| / 7\'7
| \ \   Xilinx Inc.
| / /
| \_\/.\   IBIS Models for Virtex-II
[IBIS ver]   2.1
[File name]   virtex2.ibs
[File Rev]   3.1
[Date]   6/8/04
[Source]   HSPICE simulations
[Notes]   Xilinx IBIS models for Virtex-II I/Os
These models have been verified to be an accurate representation of the
FAST/STRONG, SLOW/WEAK and TYPICAL performance corners by sample testing
of actual devices.  Actual measurements may vary, but will be well within
the performance corners if the simulation includes all other elements
that are on the printed circuit board.  These include but are not limited
to: driver, receiver(s), transmission line(s), connectors, impedance
discontinuities, and package parasitics.  Contact your Xilinx FAE or the
Xilinx Hotline for assistance.
For more information about using these IBIS models, please see
the readme file that came with this model file.
[Copyright]   Copyright 2003, Xilinx Inc., All rights reserved
|   Component Virtex-II
[Component]   Virtex-II
[Manufacturer]   Xilinx Inc.
[Package]
| variable   typ   min   max
R_pkg   0.1   NA   NA
L_pkg   0.8nH   NA   NA
C_pkg   0.5pF   NA   NA
[Pin]  signal_name   model_name   R_pin   L_pin   C_pin
|   LVTTL, fast slew rate
1   LVTTL2F   LVTTL2F
2   LVTTL4F   LVTTL4F
3   LVTTL6F   LVTTL6F
4   LVTTL8F   LVTTL8F
5   LVTTL12F   LVTTL12F
6   LVTTL16F   LVTTL16F
7   LVTTL24F   LVTTL24F
|   LVTTL, slow slew rate
8   LVTTL2S   LVTTL2S
9   LVTTL4S   LVTTL4S
10   LVTTL6S   LVTTL6S
11   LVTTL8S   LVTTL8S
12   LVTTL12S   LVTTL12S
13   LVTTL16S   LVTTL16S
14   LVTTL24S   LVTTL24S
|   LVCMOS 3.3V, fast slew rate
15   LVCM32F   LVCM32F
16   LVCM34F   LVCM34F
17   LVCM36F   LVCM36F
18   LVCM38F   LVCM38F
19   LVCM312F   LVCM312F
20   LVCM316F   LVCM316F
21   LVCM324F   LVCM324F
|   LVCMOS 3.3V, slow slew rate
22   LVCM32S   LVCM32S
23   LVCM34S   LVCM34S
24   LVCM36S   LVCM36S
25   LVCM38S   LVCM38S
26   LVCM312S   LVCM312S
27   LVCM316S   LVCM316S
28   LVCM324S   LVCM324S
|   LVCMOS 2.5V, fast slew rate
29   LVCM22F   LVCM22F
30   LVCM24F   LVCM24F
31   LVCM26F   LVCM26F
32   LVCM28F   LVCM28F
33   LVCM212F   LVCM212F
34   LVCM216F   LVCM216F
35   LVCM224F   LVCM224F
|   LVCMOS 2.5V, slow slew rate
36   LVCM22S   LVCM22S
37   LVCM24S   LVCM24S
38   LVCM26S   LVCM26S
39   LVCM28S   LVCM28S
40   LVCM212S   LVCM212S
41   LVCM216S   LVCM216S
42   LVCM224S   LVCM224S
|   LVCMOS 1.8V, fast slew rate
43   LVCM82F   LVCM82F
44   LVCM84F   LVCM84F
45   LVCM86F   LVCM86F
46   LVCM88F   LVCM88F
47   LVCM812F   LVCM812F
48   LVCM816F   LVCM816F
|   LVCMOS 1.8V, slow slew rate
49   LVCM82S   LVCM82S
50   LVCM84S   LVCM84S
51   LVCM86S   LVCM86S
52   LVCM88S   LVCM88S
53   LVCM812S   LVCM812S
54   LVCM816S   LVCM816S
|   LVCMOS 1.5V, fast slew rate
55   LVCM52F   LVCM52F
56   LVCM54F   LVCM54F
57   LVCM56F   LVCM56F
58   LVCM58F   LVCM58F
59   LVCM512F   LVCM512F
60   LVCM516F   LVCM516F
|   LVCMOS 1.5V, slow slew rate
61   LVCM52S   LVCM52S
62   LVCM54S   LVCM54S
63   LVCM56S   LVCM56S
64   LVCM58S   LVCM58S
65   LVCM512S   LVCM512S
66   LVCM516S   LVCM516S
|   HSTL 1.5V, class I-IV
67   HSTL1_15   HSTL1_15
68   HSTL2_15   HSTL2_15
69   HSTL3_15   HSTL3_15
70   HSTL4_15   HSTL4_15
|   GTL, GTLP
71   GTL   GTL
72   GTLP   GTLP
|   SSTL 1.8V, class I and II
73   SSTL18C1   SSTL18C1
74   SSTL18C2   SSTL18C2
|   SSTL2, class I and II
75   SSTL2C1   SSTL2C1
76   SSTL2C2   SSTL2C2
|   SSTL3, class I and II
77   SSTL3C1   SSTL3C1
78   SSTL3C2   SSTL3C2
|   PCI
79   PCI33   PCI33
80   PCI66   PCI66
81   PCIX   PCIX
|   AGP
82   AGP2X   AGP2X
|   LVPECL
83P   LVPECLP   LVPECL
83N   LVPECLN   LVPECL
|   LVDS 2.5V
84P   LVDS25P   LVDS25
84N   LVDS25N   LVDS25
|   LVDS 2.5V Extended
85P   LVDS25EP   LVDS25E
85N   LVDS25EN   LVDS25E
|   LVDS 3.3V
86P   LVDS33P   LVDS33
86N   LVDS33N   LVDS33
|   LVDS 3.3V Extended
87P   LVDS33EP   LVDS33E
87N   LVDS33EN   LVDS33E
|   LDT 2.5V
88P   LDT25P   LDT25
88N   LDT25N   LDT25
|   BusLVDS
89P   BUSSLVDSP   BUSSLVDS
89N   BUSSLVDSN   BUSSLVDS
|   DCI HSTL 1.5V, class I-IV, inputs
90   DCIHSTL15_I   DCIHSTL15_I
91   DCIHSTL25_I   DCIHSTL25_I
92   DCIHSTL35_I   DCIHSTL35_I
93   DCIHSTL45_I   DCIHSTL45_I
|   DCI HSTL 1.5V, class I-IV, outputs
94   DCIHSTL15_O   DCIHSTL15_O
95   DCIHSTL25_O   DCIHSTL25_O
96   DCIHSTL35_O   DCIHSTL35_O
97   DCIHSTL45_O   DCIHSTL45_O
|   DCI GTL and GTLP, inputs
98   DCIGTL_I   DCIGTL_I
99   DCIGTLP_I   DCIGTLP_I
|   DCI GTL and GTLP, outputs
100   DCIGTL_O   DCIGTL_O
101   DCIGTLP_O   DCIGTLP_O
|   DCI SSTL 1.8V, class I and II, inputs
102   DCISSTL18C1_I   DCISSTL18C1_I
103   DCISSTL18C2_I   DCISSTL18C2_I
|   DCI SSTL2, class I and II, inputs
104   DCISSTL2C1_I   DCISSTL2C1_I
105   DCISSTL2C2_I   DCISSTL2C2_I
|   DCI SSTL3, class I and II, inputs
106   DCISSTL3C1_I   DCISSTL3C1_I
107   DCISSTL3C2_I   DCISSTL3C2_I
|   DCI SSTL 1.8V, class I and II, outputs
108   DCISSTL18C1_O   DCISSTL18C1_O
109   DCISSTL18C2_O   DCISSTL18C2_O
|   DCI SSTL2, class I and II, outputs
110   DCISSTL2C1_O   DCISSTL2C1_O
111   DCISSTL2C2_O   DCISSTL2C2_O
|   DCI SSTL3, class I and II, outputs
112   DCISSTL3C1_O   DCISSTL3C1_O
113   DCISSTL3C2_O   DCISSTL3C2_O
|   DCI LVCMOS 1.5V (40, 50, 65 ohms)
114   DCILVCMOS15_40   DCILVCMOS15_40
115   DCILVCMOS15_50   DCILVCMOS15_50
116   DCILVCMOS15_65   DCILVCMOS15_65
|   DCI LVCMOS 1.8V (40, 50, 65 ohms)
117   DCILVCMOS18_40   DCILVCMOS18_40
118   DCILVCMOS18_50   DCILVCMOS18_50
119   DCILVCMOS18_65   DCILVCMOS18_65
|   DCI LVCMOS 2.5V (40, 50, 65 ohms)
120   DCILVCMOS25_40   DCILVCMOS25_40
121   DCILVCMOS25_50   DCILVCMOS25_50
122   DCILVCMOS25_65   DCILVCMOS25_65
|   DCI LVCMOS 3.3V (40, 50, 65 ohms)
123   DCILVCMOS33_40   DCILVCMOS33_40
124   DCILVCMOS33_50   DCILVCMOS33_50
125   DCILVCMOS33_65   DCILVCMOS33_65
|   DCI LVCMOS 1.5V - 3.3V, DV2 drivers
|   (*DV2_50 = 25 ohms, *DV2_65 = 32.5 ohms)
126   DCILVCMOS15DV2_50   DCILVCMOS15DV2_50
127   DCILVCMOS15DV2_65   DCILVCMOS15DV2_65
128   DCILVCMOS18DV2_50   DCILVCMOS18DV2_50
129   DCILVCMOS18DV2_65   DCILVCMOS18DV2_65
130   DCILVCMOS25DV2_50   DCILVCMOS25DV2_50
131   DCILVCMOS25DV2_65   DCILVCMOS25DV2_65
132   DCILVCMOS33DV2_50   DCILVCMOS33DV2_50
133   DCILVCMOS33DV2_65   DCILVCMOS33DV2_65
|   HSTL 1.8V, class I-IV
134   HSTL1_18   HSTL1_18
135   HSTL2_18   HSTL2_18
136   HSTL3_18   HSTL3_18
137   HSTL4_18   HSTL4_18
|   DCI HSTL 1.8V, class I-IV, inputs
138   DCIHSTL18_I   DCIHSTL18_I
139   DCIHSTL28_I   DCIHSTL28_I
140   DCIHSTL38_I   DCIHSTL38_I
141   DCIHSTL48_I   DCIHSTL48_I
|   DCI HSTL 1.8V, class I-IV, outputs
142   DCIHSTL18_O   DCIHSTL18_O
143   DCIHSTL28_O   DCIHSTL28_O
144   DCIHSTL38_O   DCIHSTL38_O
145   DCIHSTL48_O   DCIHSTL48_O
|   LVDS 2.5V input, DCI-controlled termination
146   DCILVDS25   DCILVDS25
|   High-Speed LVDCI (1.8V DCI LVCMOS driver, HSTL1 receiver)
|   40, 50, 65 ohms
|   *DV2_50 = 25 ohms, *DV2_65 = 32.5 ohms
147   HSLVDCI_18_40   HSLVDCI_18_40
148   HSLVDCI_18_50   HSLVDCI_18_50
149   HSLVDCI_18_65   HSLVDCI_18_65
150   HSLVDCI_18_DV2_50   HSLVDCI_18_DV2_50
151   HSLVDCI_18_DV2_65   HSLVDCI_18_DV2_65
PGND   GND   GND
VCCO   VCCO   POWER
[Diff Pin]   inv_pin   vdiff   tdelay_typ   tdelay_min   tdelay_max
| Here is just a sample format for differential pin pairs.
| Edit the list based on your applications.
83P   83N   850mV   0   0   0
84P   84N   350mV   0   0   0
85P   85N   630mV   0   0   0
86P   86N   350mV   0   0   0
87P   87N   630mV   0   0   0
88P   88N   600mV   0   0   0
89P   89N   350mV   0   0   0
| Models and submodels in the file (151): LVTTL2F (I/O), LVTTL4F (I/O), LVTTL6F (I/O), LVTTL8F (I/O), LVTTL12F (I/O), LVTTL16F (I/O), LVTTL24F (I/O), LVTTL2S (I/O), LVTTL4S (I/O), LVTTL6S (I/O), LVTTL8S (I/O), LVTTL12S (I/O), LVTTL16S (I/O), LVTTL24S (I/O), LVCM32F (I/O), LVCM34F (I/O), LVCM36F (I/O), LVCM38F (I/O), LVCM312F (I/O), LVCM316F (I/O), LVCM324F (I/O), LVCM32S (I/O), LVCM34S (I/O), LVCM36S (I/O), LVCM38S (I/O), LVCM312S (I/O), LVCM316S (I/O), LVCM324S (I/O), LVCM22F (I/O), LVCM24F (I/O), LVCM26F (I/O), LVCM28F (I/O), LVCM212F (I/O), LVCM216F (I/O), LVCM224F (I/O), LVCM22S (I/O), LVCM24S (I/O), LVCM26S (I/O), LVCM28S (I/O), LVCM212S (I/O), LVCM216S (I/O), LVCM224S (I/O), LVCM82F (I/O), LVCM84F (I/O), LVCM86F (I/O), LVCM88F (I/O), LVCM812F (I/O), LVCM816F (I/O), LVCM82S (I/O), LVCM84S (I/O), LVCM86S (I/O), LVCM88S (I/O), LVCM812S (I/O), LVCM816S (I/O), LVCM52F (I/O), LVCM54F (I/O), LVCM56F (I/O), LVCM58F (I/O), LVCM512F (I/O), LVCM516F (I/O), LVCM52S (I/O), LVCM54S (I/O), LVCM56S (I/O), LVCM58S (I/O), LVCM512S (I/O), LVCM516S (I/O), HSTL1_15 (I/O), HSTL2_15 (I/O), HSTL3_15 (I/O), HSTL4_15 (I/O), GTL (I/O_open_drain), GTLP (I/O_open_drain), SSTL18C1 (I/O), SSTL18C2 (I/O), SSTL2C1 (I/O), SSTL2C2 (I/O), SSTL3C1 (I/O), SSTL3C2 (I/O), PCI33 (I/O), PCI66 (I/O)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
